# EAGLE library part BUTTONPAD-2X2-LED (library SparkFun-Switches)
2x2 Button Pad w/ Single LEDs Layout and schematic for 2x2 button pad with single-color LEDs under each button. For use with the Button Pad 2x2 - LED Compatible and Button Pad 2x2 Top Bezel. Any single-color 5mm LED should be compatible. SparkFun Products SparkFun Simon Says - Through-Hole Soldering Kit (KIT-10547) Button Pad 2x2 - Breakout PCB (COM-09277)
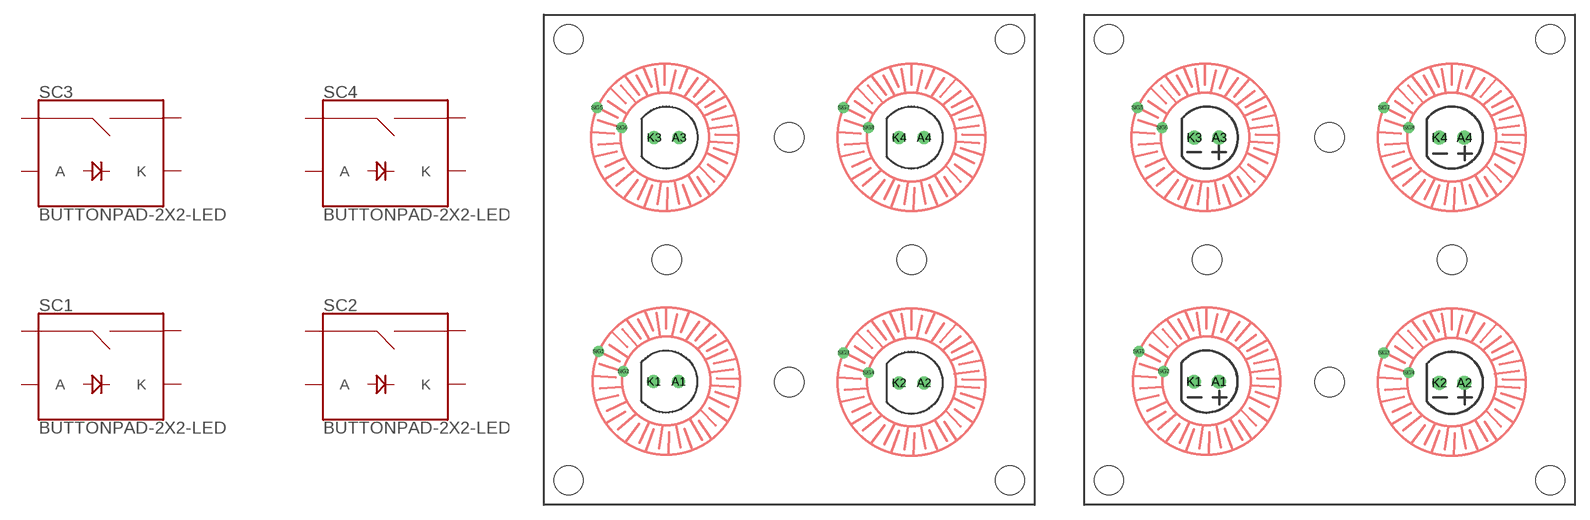
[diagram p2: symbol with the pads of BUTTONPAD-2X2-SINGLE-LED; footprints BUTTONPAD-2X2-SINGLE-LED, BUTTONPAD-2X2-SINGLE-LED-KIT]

Designator prefix S; gates C1=BUTTONPAD-LED C2=BUTTONPAD-LED C3=BUTTONPAD-LED C4=BUTTONPAD-LED

## BUTTONPAD-2X2-LED (PROD_ID: COMP-08481; SF_SKU: COM-07836)  [BUTTONPAD-2X2-SINGLE-LED]
A1  C1:A
A2  C2:A
A3  C3:A
A4  C4:A
K1  C1:K
K2  C2:K
K3  C3:K
K4  C4:K
SIG1  C1:SIG1
SIG2  C1:SIG2
SIG3  C2:SIG1
SIG4  C2:SIG2
SIG5  C3:SIG1
SIG6  C3:SIG2
SIG7  C4:SIG1
SIG8  C4:SIG2

## BUTTONPAD-2X2-LEDKIT (PROD_ID: COMP-08481; SF_SKU: COM-07836)  [BUTTONPAD-2X2-SINGLE-LED-KIT]
Pads as for BUTTONPAD-2X2-SINGLE-LED

## Footprint BUTTONPAD-2X2-SINGLE-LED (pad centres in mm)
2x2 Button Pad w/ Single LEDs Layout and schematic for 2x2 button pad with single-color LEDs under each button. For use with the Button Pad 2x2 - LED Compatible and Button Pad 2x2 Top Bezel. Any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
drill 0.813: A1 13.716,12.573; A2 38.735,12.446; A3 13.75,37.47; A4 38.735,37.465; K1 11.176,12.573; K2 36.195,12.446; K3 11.21,37.47; K4 36.195,37.465
drill 0.6: SIG1 5.542,15.64; SIG2 8.082,13.608; SIG3 30.542,15.513; SIG4 33.082,13.481; SIG5 5.388,40.513; SIG6 7.928,38.481; SIG7 30.542,40.513; SIG8 33.082,38.481
hole 3 at 12.5,25
hole 3 at 25,37.5
hole 3 at 37.5,25
hole 3 at 25,12.5
hole 3 at 2.5,2.5
hole 3 at 2.5,47.5
hole 3 at 47.5,47.5
hole 3 at 47.5,2.5

## Footprint BUTTONPAD-2X2-SINGLE-LED-KIT (pad centres in mm)
2x2 Button Pad w/ Single LEDs Layout and schematic for 2x2 button pad with single-color LEDs under each button. For use with the Button Pad 2x2 - LED Compatible and Button Pad 2x2 Top Bezel. Any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
drill 0.889 pad 1.016: A1 13.716,12.573; A2 38.735,12.446; A3 13.75,37.47; A4 38.735,37.465; K1 11.176,12.573; K2 36.195,12.446; K3 11.21,37.47; K4 36.195,37.465
drill 0.6: SIG1 5.542,15.64; SIG2 8.082,13.608; SIG3 30.542,15.513; SIG4 33.082,13.481; SIG5 5.388,40.513; SIG6 7.928,38.481; SIG7 30.542,40.513; SIG8 33.082,38.481
hole 3 at 12.5,25
hole 3 at 25,37.5
hole 3 at 37.5,25
hole 3 at 25,12.5
hole 3 at 2.5,2.5
hole 3 at 2.5,47.5
hole 3 at 47.5,47.5
hole 3 at 47.5,2.5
